FUNCTION_BLOCK "IMAC_MOTOR3"
TITLE = MOTOR 3
//--------------------------------------------------------------------------------
//SIEMENS AG     I&S IP PEP SN                        PSP-Element: D-09300081-E-E5
//--------------------------------------------------------------------------------
//History
//=======
//Date      Version  Description                        Author
//1997/06/09   0.6   Basic Edition                      Salge
//2004/11/05   1.0   Basic Edition converted to S7      Edelmann
//2004/12/07   1.1   Interface adapted                  Edelmann
//2004/12/07   1.1   Reset Outputs with feedbacks       Edelmann
//
//--------------------------------------------------------------------------------
//PLC:   >= S7-300
//--------------------------------------------------------------------------------
//Specification:   Refer "TECHFUNK.DOC"
//--------------------------------------------------------------------------------
//
//--------------------------------------------------------------------------------
//Called FC: FC90 "DELAYTIMER"
//           SFC20 "BLKMOV"
//--------------------------------------------------------------------------------
//
//--------------------------------------------------------------------------------
//Note:
//--------------------------------------------------------------------------------
// KNOW_HOW_PROTECT
AUTHOR : Sa_Edm
FAMILY : IMAC
NAME : Motor3
VERSION : 1.1


VAR_INPUT
  OBJ : INT ;
  RMOT : BOOL ;	//Local / Remote
  FWD : BOOL ;
  BACK : BOOL ;
  SLOW : BOOL ;
  FAST : BOOL ;
  FAUL : BOOL ;
  ACOM : WORD ;
  BLKO : BOOL ;
  PCONF : STRUCT
   LastRecord : INT  := 100;
   Pointer1stRecord : STRUCT
    S7ID : BYTE  := B#16#10;	//ANY pointer: ID S7
    RepeatFactor : INT  := 104;	//ANY pointer: repeat factor
    Typ : BYTE  := B#16#2;	//ANY pointer: data typ =02 BYTE =04 WORD =05 INT =06 DWORD =07 DINT =08 REAL
    DBNo : INT  := 82;	//ANY pointer: DB number, zero if no DB
    MemoryArea : BYTE  := B#16#84;	//ANY pointer: Memory area =81 IN =82 OUT =83 M =84 DB =85 DI =86 L
    DWHigh : BYTE ;	//ANY pointer: DW highest byte
    DWX : INT ;	//ANY pointer: DW low / bit (address = byte *8 + bit)
   END_STRUCT ;
  END_STRUCT ;
END_VAR
VAR_OUTPUT
  MFWD : BOOL ;
  MBAC : BOOL ;
  MSLO : BOOL ;
  MFAS : BOOL ;
  MSTO : BOOL ;
  STAT : WORD ;
  OSSTAT : WORD ;	//Status for OS
  OSALARM : WORD ;	//Alarms for OS
END_VAR
VAR_IN_OUT
  OSCOM : WORD ;
END_VAR
VAR
  Motor3 : STRUCT
   System : WORD ;
   CmdOS : WORD ;
   MirrorCmdOS : WORD ;
   Test : WORD ;
   AlarmOS : WORD ;
   StatusOS : WORD ;
   SysStatusOS : WORD ;
   Status1 : WORD ;
   Status2 : WORD ;
   Status3 : BYTE ;
   InputEdges : BYTE ;
   AutoEdges : WORD ;
   DataTimeExtFault : STRUCT
    StartTime : DINT ;
    StartEdge : BOOL ;
   END_STRUCT ;
   DataTimeFeedback : STRUCT
    StartTime : DINT ;
    StartEdge : BOOL ;
   END_STRUCT ;
   DataTimeActFault : STRUCT
    StartTime : DINT ;
    StartEdge : BOOL ;
   END_STRUCT ;
   DataTimeAutoAl : STRUCT
    StartTime : DINT ;
    StartEdge : BOOL ;
   END_STRUCT ;
   DataTimeRestart : STRUCT
    StartTime : DINT ;
    StartEdge : BOOL ;
   END_STRUCT ;
   DataTimeChgSF : STRUCT
    StartTime : DINT ;
    StartEdge : BOOL ;
   END_STRUCT ;
   DataTimeChgFS : STRUCT
    StartTime : DINT ;
    StartEdge : BOOL ;
   END_STRUCT ;
   DataTimeChgDirec : STRUCT
    StartTime : DINT ;
    StartEdge : BOOL ;
   END_STRUCT ;
   PCONF : STRUCT
    Modeswitches : STRUCT
     M0_ConstantOut : BOOL ;	// Constant Output MST1 MST2 MSTO (1); Feedback depended Output Anst. (0)
     M1_AutoManLoc : BOOL ;	// AUTO/ MANUAL/ LOCAL (1); MANUAL/ LOCAL (0)
     M2_NoActFeedFault : BOOL ;	// No Action- and Non-Feedback fault(1),
     M3_NoStopIfFault : BOOL ;	// No Stop-Signal if Failure occurs (1)
     M4_RestrtAftBlack : BOOL ;	// Restart after Blackout (1)
     M5_ResetOSonly : BOOL ;	// Reset Alarm only with RESET from OS (1); RESET and START/STOP-Command (0)
     sw06 : BOOL ;
     M7_ChgSFviaStop : BOOL ;	// Change from Slow->Fast via STOP(1)
     M8_ChgFSviaStop : BOOL ;	// Change from Fast->Slow via STOP(1)
     M9_StopIfAutoFail : BOOL ;	// Direct Stop if Auto Failure (1)
     M10_ExtFaultNC : BOOL ;
     sw11 : BOOL ;
     sw12 : BOOL ;
     sw13 : BOOL ;
     sw14 : BOOL ;
     sw15 : BOOL ;	//
    END_STRUCT ;
    DlyTExtFault : TIME ;	// Setpoint external fault delay
    DlyTFeedback : TIME ;	// Setpoint feedback fault delay
    DlyTActFault : TIME ;	// Setpoint Action Fault delay
    DlyTAutoAl : TIME ;	// Setpoint auto alarm delay
    DlyTRestart : TIME ;	// Setpoint restart after blackout delay
    DlyTChgSF : TIME ;	// Setpoint Waiting Delay Slow->Fast
    DlyTChgFS : TIME ;	// Setpoint Waiting Delay Fast->Slow
    DlyTChgDirec : TIME ;	// Setpoint change direction
   END_STRUCT ;
  END_STRUCT ;
  siFailRR : INT ;	//Failure blockmove read record
  siFailWR : INT ;	//Failure blockmove write record
END_VAR
VAR_TEMP
  M_200_0 : BOOL ;
  tbCmdManual : BOOL ;
  tbCmdAuto : BOOL ;
  M_200_3 : BOOL ;
  M_200_4 : BOOL ;
  M_200_5 : BOOL ;
  M_200_6 : BOOL ;
  M_200_7 : BOOL ;
  tbCmdStartR1 : BOOL ;
  tbCmdStartR2 : BOOL ;
  tbCmdStartL1 : BOOL ;
  tbCmdStartL2 : BOOL ;
  tbCmdStop : BOOL ;
  M_201_5 : BOOL ;
  M_201_6 : BOOL ;
  tbCmdReset : BOOL ;
  M_202_0 : BOOL ;
  M_202_1 : BOOL ;
  M_202_2 : BOOL ;
  M_202_3 : BOOL ;
  M_202_4 : BOOL ;
  M_202_5 : BOOL ;
  M_202_6 : BOOL ;
  M_202_7 : BOOL ;
  M_203_0 : BOOL ;
  M_203_1 : BOOL ;
  tbAutoFailInput : BOOL ;
  tbCmdLock : BOOL ;
  tbEmergencyOff : BOOL ;
  M_203_5 : BOOL ;
  M_203_6 : BOOL ;
  M_203_7 : BOOL ;
  M_204_0 : BOOL ;
  M_204_1 : BOOL ;
  M_204_2 : BOOL ;
  M_204_3 : BOOL ;
  M_204_4 : BOOL ;
  M_204_5 : BOOL ;
  M_204_6 : BOOL ;
  M_204_7 : BOOL ;
  tbCommandStartR1Auto : BOOL ;
  tbCommandStopAuto : BOOL ;
  tbAutoFailInputPulse : BOOL ;
  M_205_3 : BOOL ;
  M_205_4 : BOOL ;
  tbCommandStartR2Auto : BOOL ;
  tbCommandStartL1Auto : BOOL ;
  tbCommandStartL2Auto : BOOL ;
  tbRemoteLocal : BOOL ;
  tbRunningFWD : BOOL ;
  tbFault : BOOL ;
  tbBlackout : BOOL ;
  tbRunningBack : BOOL ;
  tbRunningSlow : BOOL ;
  tbRunningFast : BOOL ;
  M_206_7 : BOOL ;
  M_207_0 : BOOL ;
  M_207_1 : BOOL ;
  M_207_2 : BOOL ;
  M_207_3 : BOOL ;
  M_207_4 : BOOL ;
  M_207_5 : BOOL ;
  M_207_6 : BOOL ;
  M_207_7 : BOOL ;
  tbStateFWDFast : BOOL ;
  tbStateBackSlow : BOOL ;
  tbStateBackFast : BOOL ;
  M_208_3 : BOOL ;
  M_208_4 : BOOL ;
  M_208_5 : BOOL ;
  M_208_6 : BOOL ;
  M_208_7 : BOOL ;
  tbStateFWDSlow : BOOL ;
  tbStateLocal : BOOL ;
  tbStateManual : BOOL ;
  tbStateAuto : BOOL ;
  tbStateFault : BOOL ;
  tbStateBlackout : BOOL ;
  M_209_6 : BOOL ;
  M_209_7 : BOOL ;
  M_210_0 : BOOL ;
  M_210_1 : BOOL ;
  M_210_2 : BOOL ;
  M_210_3 : BOOL ;
  M_210_4 : BOOL ;
  M_210_5 : BOOL ;
  M_210_6 : BOOL ;
  M_210_7 : BOOL ;
  M_211_0 : BOOL ;
  M_211_1 : BOOL ;
  M_211_2 : BOOL ;
  M_211_3 : BOOL ;
  M_211_4 : BOOL ;
  M_211_5 : BOOL ;
  M_211_6 : BOOL ;
  M_211_7 : BOOL ;
  M_212_0 : BOOL ;
  M_212_1 : BOOL ;
  M_212_2 : BOOL ;
  M_212_3 : BOOL ;
  M_212_4 : BOOL ;
  M_212_5 : BOOL ;
  M_212_6 : BOOL ;
  M_212_7 : BOOL ;
  M_213_0 : BOOL ;
  M_213_1 : BOOL ;
  M_213_2 : BOOL ;
  M_213_3 : BOOL ;
  M_213_4 : BOOL ;
  M_213_5 : BOOL ;
  M_213_6 : BOOL ;
  M_213_7 : BOOL ;
  tbNonFeedbackTimer : BOOL ;
  tbNonFeedbackAlarm : BOOL ;
  tbActionTimer : BOOL ;
  tbActionAlarm : BOOL ;
  tbAutoTimer : BOOL ;
  tbAutoAlarm : BOOL ;
  tbBlackoutStartF1 : BOOL ;
  tbRestartAfterBlackout : BOOL ;
  tbOutStartF1 : BOOL ;
  tbOutStop : BOOL ;
  tbLocal : BOOL ;
  tbOutManual : BOOL ;
  tbOutAuto : BOOL ;
  M_215_5 : BOOL ;
  tbExternalFault : BOOL ;
  tbFaultInputAlarm : BOOL ;
  tbBlackoutStartB1 : BOOL ;
  tbOutStartB2 : BOOL ;
  tbBlackoutStartB2 : BOOL ;
  tbOutputMFWD : BOOL ;
  tbOutputMBAC : BOOL ;
  tbOutputMSLO : BOOL ;
  tbOutputMFAS : BOOL ;
  tbOutputMSTO : BOOL ;
  M_217_0 : BOOL ;
  tbOutChangeToStartF1 : BOOL ;
  tbOutChangeToStartF2 : BOOL ;
  tbOutChangeToStartB1 : BOOL ;
  tbOutChangeToStartB2 : BOOL ;
  tbOutStartF2 : BOOL ;
  tbBlackoutStartF2 : BOOL ;
  tbOutStartB1 : BOOL ;
  tbLocaltoRemote : BOOL ;
  M_218_1 : BOOL ;
  M_218_2 : BOOL ;
  M_218_3 : BOOL ;
  M_218_4 : BOOL ;
  M_218_5 : BOOL ;
  M_218_6 : BOOL ;
  M_218_7 : BOOL ;
  tbWaitingTime1_2 : BOOL ;
  tbWaitingTime2_1 : BOOL ;
  tbChangeDirecTimer2_1 : BOOL ;
  M_219_3 : BOOL ;
  tbResetStopping : BOOL ;
  M_219_5 : BOOL ;
  M_219_6 : BOOL ;
  M_219_7 : BOOL ;
  M_220_0 : BOOL ;
  M_220_1 : BOOL ;
  M_220_2 : BOOL ;
  M_220_3 : BOOL ;
  M_220_4 : BOOL ;
  M_220_5 : BOOL ;
  M_220_6 : BOOL ;
  M_220_7 : BOOL ;
  M_221_0 : BOOL ;
  M_221_1 : BOOL ;
  M_221_2 : BOOL ;
  M_221_3 : BOOL ;
  M_221_4 : BOOL ;
  M_221_5 : BOOL ;
  M_221_6 : BOOL ;
  M_221_7 : BOOL ;
  P_currentRecord : ANY ;	//ANY pointer of the current record
END_VAR
BEGIN
NETWORK
TITLE =Calculation of current ANY pointer for reading /writing record
// ANY-pointer of current record
      L     #PCONF.Pointer1stRecord.S7ID;
      T     LB    22;
      L     #PCONF.Pointer1stRecord.Typ;
      T     LB    23;
      L     #PCONF.Pointer1stRecord.RepeatFactor;
      T     LW    24;
      L     #PCONF.Pointer1stRecord.DBNo;
      T     LW    26;
      L     #PCONF.Pointer1stRecord.MemoryArea;
      T     LB    28;
      L     #PCONF.Pointer1stRecord.DWHigh;
      T     LB    29;
      L     #PCONF.Pointer1stRecord.DWX;
      T     LW    30;

      L     #OBJ; //Check whether Obj within the range
      L     #PCONF.LastRecord;
      >I    ;
      SPB   cRcd;
      L     #OBJ;
      L     1;
      <I    ;
      SPB   cRcd;
      L     #OBJ;
cRcd: +     -1;
      L     #PCONF.Pointer1stRecord.RepeatFactor;
      *I    ;
      SLD   3; //DBW + DBX address of the current record
      L     LD    28;
      OD    ;
      T     LD    28; //DBWX part of ANY pointer "P_currentRecord"
NETWORK
TITLE =Read record

      CALL "BLKMOV" (
           SRCBLK                   := #P_currentRecord,
           RET_VAL                  := #siFailRR,
           DSTBLK                   := #Motor3);

NETWORK
TITLE =Read OS command

      L     #OSCOM; // Commands from OS
      T     LW     0;
      L     #Motor3.Status1; // Status stored
      T     LW    14;
      L     #Motor3.Status2; // Status stored
      T     LW    16;
      L     #Motor3.Status3; // Status stored
      T     LB    19;

      L     0; //Reset scratch  flags
      T     LW     6;
      T     LW    50;
      T     LW    52;
      T     LW    54;
NETWORK
TITLE =Formaloperanden Inputs

      U     #RMOT;
      =     #tbRemoteLocal; //Remote/Local
      U     #FWD;
      =     #tbRunningFWD; //Running foreward
      U     #BACK;
      =     #tbRunningBack; //Running back
      U     #SLOW;
      =     #tbRunningSlow; //Running slow
      U     #FAST;
      =     #tbRunningFast; //Running fast

      U     #Motor3.PCONF.Modeswitches.M10_ExtFaultNC;
      SPB   NC;
      U     #FAUL;
      =     #tbFault; //Fault
      SPA   GO;
NC:   UN    #FAUL;
      =     #tbFault; //Fault

GO:   L     #ACOM;
      T     LW     2; // Command From Automatic

      U     #BLKO;
      =     #tbBlackout; //Blackout

// ----Evaluate Pulsflags from Auto Commands----
      L     #Motor3.AutoEdges; //Stored Auto Command last cycle
      INVI  ; //Singlecomplement
      L     LW     2; //Command From Automatic
      T     #Motor3.AutoEdges;
      UW    ;
      T     LW     4; // Command  Pulseflags

// ----Evaluate Pulsflags from Inputs----
      L     #Motor3.InputEdges; //Stored Auto Command last cycle
      INVI  ; //Singlecomplement
      L     LB     6; //Inputs
      T     #Motor3.InputEdges;
      UW    ;
      T     LB    18; // Inputs Pulseflags
NETWORK
TITLE =Local-Manual- Auto

      UN    #tbRemoteLocal; // Not Remote
      =     #tbLocal; // LOCAL
      R     #tbOutManual; // MANUAL!
      R     #tbOutAuto; // AUTO!
      R     #tbOutChangeToStartF1; // Change to STARTF1!
      R     #tbOutChangeToStartF2; // Change to STARTF2!
      R     #tbOutChangeToStartB1; // Change to STARTB1!
      R     #tbOutChangeToStartB2; // Change to STARTB2!
      R     #tbOutStartF1; // STARTF1!
      R     #tbOutStartF2; // STARTF2!
      R     #tbOutStartB1; // STARTB1!
      R     #tbOutStartB2; // STARTB2!
      R     #tbOutStop; // STOP!
      R     #tbBlackoutStartF1; // BLACKOUT START F1
      R     #tbBlackoutStartF2; // BLACKOUT START F2
      R     #tbBlackoutStartB1; // BLACKOUT START B1
      R     #tbBlackoutStartB2; // BLACKOUT START B2
      R     #tbNonFeedbackTimer; // reset Non Feedback Timer
      R     #tbActionTimer; // reset Action Timer
      R     #tbAutoTimer; // reset Auto Timer
      R     #tbWaitingTime1_2; // reset Wating timer1->2
      R     #tbChangeDirecTimer2_1; // Change direction timer2->1
      R     #tbResetStopping; // reset Stopping


      SPB   E05;
      U     #Motor3.PCONF.Modeswitches.M1_AutoManLoc; // extra Automode ?
      SPB   MODE;
      S     #tbOutManual; //MANUAL!
      S     #tbOutAuto; // AUTO!
      SPA   E05;
MODE: U     #tbCmdManual; //Command Manual
      S     #tbOutManual; //MANUAL!
      R     #tbOutAuto; // AUTO!
      U     #tbCmdAuto; //Command Auto
      S     #tbOutAuto; // AUTO!
      R     #tbOutManual; // MANUAL!
      UN    #tbOutAuto; // AUTO!
      UN    #tbOutManual; // MANUAL!
      S     #tbOutManual; // MANUAL!
E05:  NOP   0;


NETWORK
TITLE =Commands
// SET Start forward 1 Command
      L     LW     0;
      U     #M_200_7;
      U     #tbCmdReset;
      O(    ;
      U     #tbCmdStartR1; //Command Start R1  OS Pulse
      U     #tbOutManual; //MANUAL!
      )     ;
      O(    ;
      U     #tbCommandStartR1Auto; //Command Start R1 Auto Pulse
      U     #tbOutAuto; //AUTO!
      )     ;
      S     #tbOutStartF1; //STARTF1!
      S     L     51.0; //STARTF1 Pulse

//SET Start Forward 2 Command
      O(    ;
      U     #tbCmdStartR2; //Command Start R2 OS Pulse
      U     #tbOutManual; //MANUAL!
      )     ;
      O(    ;
      U     #tbCommandStartR2Auto; //Command Start R2 Auto Pulse
      U     #tbOutAuto; //AUTO!
      )     ;
      S     #tbOutStartF2; //STARTF2!
      S     L     51.2; //STARTF2 Pulse

//SET Start BACK1 Command
      O(    ;
      U     #tbCmdStartL1; //Command Start L1  OS Pulse
      U     #tbOutManual; //MANUAL!
      )     ;
      O(    ;
      U     #tbCommandStartL1Auto; //Command Start L1 Auto Pulse
      U     #tbOutAuto; //AUTO!
      )     ;
      S     #tbOutStartB1; //STARTB1!
      S     L     51.3; //STARTF1 Pulse

//SET Start Back2 Command
      O(    ;
      U     #tbCmdStartL2; //Command Start L2 OS Pulse
      U     #tbOutManual; //MANUAL!
      )     ;
      O(    ;
      U     #tbCommandStartL2Auto; //Command Start L2 Auto Pulse | Corr: Edm, 08.12.04
      U     #tbOutAuto; //AUTO!
      )     ;
      S     #tbOutStartB2; //STARTB2!
      S     L     51.4; //STARTB2 Pulse

//SET Stop Command
      O(    ;
      U     #tbCmdStop; //Command Stop OS Pulse
      U     #tbOutManual; //MANUAL!
      )     ;
      O(    ;
      U     #tbCommandStopAuto; //Command Stop Auto Pulse
      U     #tbOutAuto; //AUTO!
      )     ;
      S     #tbOutStop; //STOP!
      S     L     51.1; //STOP Pulse
      R     #tbOutChangeToStartF1; //Change to STARTF1!
      R     #tbOutChangeToStartF2; //Change to STARTF2!
      R     #tbOutChangeToStartB1; //Change to STARTB1!
      R     #tbOutChangeToStartB2; //Change to STARTB2!

//Reset Alarms
      O     L     51.0; //STARTF1! Pulse
      O     L     51.2; //STARTF2! Pulse
      O     L     51.3; //STARTB1! Pulse
      O     L     51.4; //STARTB2! Pulse
      O     L     51.1; //STOP! Pulse
      U     #Motor3.PCONF.Modeswitches.M5_ResetOSonly; //Modeswitch Reset Alarm with Start/Stop
      O     #tbCmdReset; //Command RESET OS Pulse
      R     #tbFaultInputAlarm; //Fault Input Alarm
      R     #tbNonFeedbackAlarm; //Non Feedback Alarm
      R     #tbActionAlarm; //Action Alarm
      R     #tbActionTimer; //Edm, 08.12.04
      R     #tbAutoAlarm; //Auto Alarm

//Reset START ! if Failure
      O     #tbFaultInputAlarm; //Fault Input Alarm
      O     #tbNonFeedbackAlarm; //Non Feedback Alarm
      O     #tbActionAlarm; //Action Alarm
      O     #tbAutoAlarm; //Auto Alarm
      U     #tbOutStartF1; //STARTF1!
      U     L     51.0; //STARTF1 Pulse
      R     #tbOutStartF1; //STARTF1!
      R     L     51.0; //STARTF1 Pulse
      S     #tbOutStop; //STOP!

      O     #tbFaultInputAlarm; //Fault Input Alarm
      O     #tbNonFeedbackAlarm; //Non Feedback Alarm
      O     #tbActionAlarm; //Action Alarm
      O     #tbAutoAlarm; //Auto Alarm
      U     #tbOutStartF2; //STARTF2
      U     L     51.2; //STARTF2 Pulse
      R     #tbOutStartF2; //STARTF2
      R     L     51.2; //STARTF2 Pulse
      S     #tbOutStop; //STOP!

      O     #tbFaultInputAlarm; //Fault Input Alarm
      O     #tbNonFeedbackAlarm; //Non Feedback Alarm
      O     #tbActionAlarm; //Action Alarm
      O     #tbAutoAlarm; //Auto Alarm
      U     #tbOutStartB1; //STARTB1!
      U     L     51.3; //STARTB1 Pulse
      R     #tbOutStartB1; //STARTB1!
      R     L     51.3; //STARTB1 Pulse
      S     #tbOutStop; //STOP!

      O     #tbFaultInputAlarm; //Fault Input Alarm
      O     #tbNonFeedbackAlarm; //Non Feedback Alarm
      O     #tbActionAlarm; //Action Alarm
      O     #tbAutoAlarm; //Auto Alarm
      U     #tbOutStartB2; //STARTB2!
      U     L     51.4; //STARTB2 Pulse
      R     #tbOutStartB2; //STARTB2!
      R     L     51.4; //STARTB2 Pulse
      S     #tbOutStop; //STOP!

      U     #tbLocaltoRemote; //Local to Remote Pulse
      U     #tbRunningFWD; //Running foreward
      U     #tbRunningSlow; //Running slow
      UN    #tbOutStartF1; //STARTF1!
      UN    #tbOutStartF2; //STARTF2!
      UN    #tbOutStartB1; //STARTB1!
      UN    #tbOutStartB2; //STARTB2!
      UN    #tbOutStop; //STOP!
      S     #tbOutStartF1; //STARTF1!

      U     #tbLocaltoRemote; //Local to Remote Pulse
      U     #tbRunningFWD; //Running foreward
      U     #tbRunningFast; //Running fast
      UN    #tbOutStartF1; //STARTF1!
      UN    #tbOutStartF2; //STARTF2!
      UN    #tbOutStartB1; //STARTB1!
      UN    #tbOutStartB2; //STARTB2!
      UN    #tbOutStop; //STOP!
      S     #tbOutStartF2; //STARTF2!

      U     #tbLocaltoRemote; //Local to Remote Pulse
      U     #tbRunningBack; //Running back
      U     #tbRunningSlow; //Running slow
      UN    #tbOutStartF1; //STARTF1!
      UN    #tbOutStartF2; //STARTF2!
      UN    #tbOutStartB1; //STARTB1!
      UN    #tbOutStartB2; //STARTB2!
      UN    #tbOutStop; //STOP!
      S     #tbOutStartB1; //STARTB1!

      U     #tbLocaltoRemote; //Local to Remote Pulse
      U     #tbRunningBack; //Running back
      U     #tbRunningFast; //Running fast
      UN    #tbOutStartF1; //STARTF1!
      UN    #tbOutStartF2; //STARTF2!
      UN    #tbOutStartB1; //STARTB1!
      UN    #tbOutStartB2; //STARTB2!
      UN    #tbOutStop; //STOP!
      S     #tbOutStartB2; //STARTB2!
NETWORK
TITLE =Change Mode 1
//STOP F1,F2,B1,B2 after 0
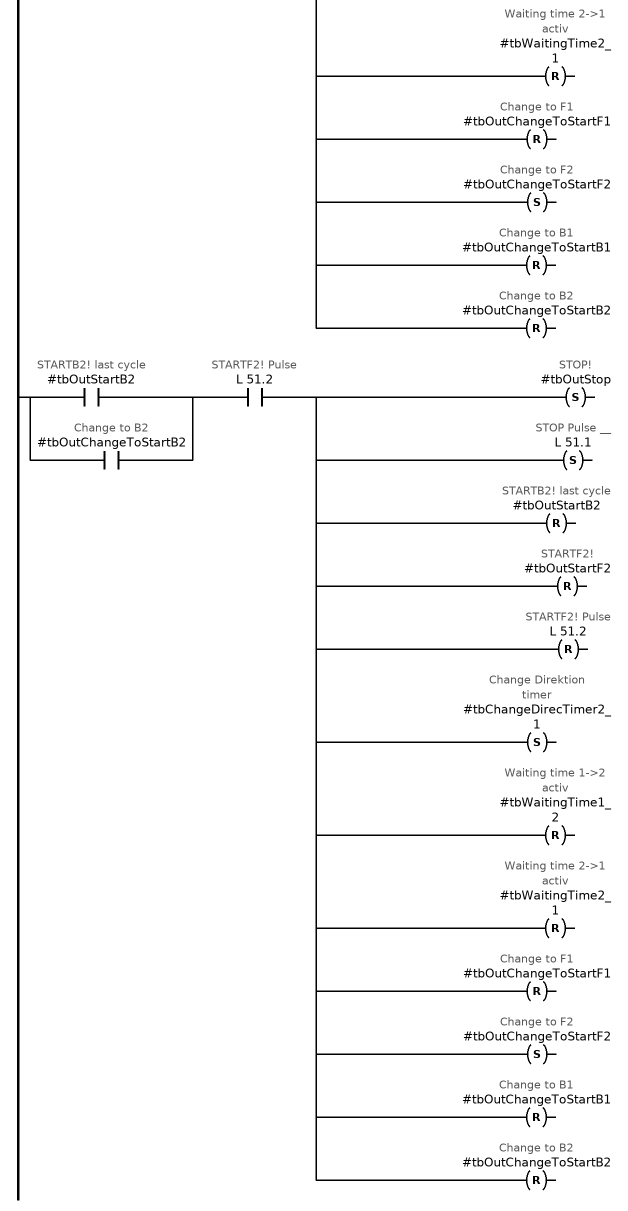
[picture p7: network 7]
      O     #tbOutStartF1; //STARTF1! Last cycle
      O     #tbOutStartF2; //STARTF2! Last cycle
      O     #tbOutStartB1; //STARTB1! Last cycle
      O     #tbOutStartB2; //STARTB2! Last cycle
      U     L     51.1; //STOP Pulse
      S     #tbChangeDirecTimer2_1; //Change Direktion timer
      R     #tbWaitingTime2_1; //Waiting time 2->1 activ
      R     #tbWaitingTime1_2; //Waiting time 1->2 activ

//Change from F1 to F2
      U     #tbOutStartF1; //STARTF1! last cycle
      U     L     51.2; //STARTF2! Pulse
      U     #Motor3.PCONF.Modeswitches.M7_ChgSFviaStop; //MOD Change from 1->2 via Stop
      S     #tbOutStop; //STOP!
      S     L     51.1; //STOP Pulse

      U     #tbOutStartF1; //STARTF1! last cycle
      U     L     51.2; //STARTF2! Pulse
      R     #tbOutStartF1; //STARTF1! last cycle
      R     #tbOutStartF2; //STARTF2!
      R     L     51.2; //STARTF2! Pulse
      S     #tbChangeDirecTimer2_1; //Change Direktion timer
      S     #tbWaitingTime1_2; //Waiting time 1->2 activ
      R     #tbWaitingTime2_1; //Waiting time 2->1 activ
      R     #tbOutChangeToStartF1; //Change to F1
      S     #tbOutChangeToStartF2; //Change to F2
      R     #tbOutChangeToStartB1; //Change to B1
      R     #tbOutChangeToStartB2; //Change to B2

//Change from F2 to F1
      U     #tbOutStartF2; //STARTF2! last cycle
      U     L     51.0; //STARTF1! Pulse
      U     #Motor3.PCONF.Modeswitches.M8_ChgFSviaStop; //MOD Change from 2->1 via Stop
      S     #tbOutStop; //STOP!
      S     L     51.1; //STOP Pulse

      U     #tbOutStartF2; //STARTF2! last cycle
      U     L     51.0; //STARTF1! Pulse
      R     #tbOutStartF2; //STARTF2! last cycle
      R     #tbOutStartF1; //STARTF1! _
      R     L     51.0; //STARTF1! Pulse
      S     #tbChangeDirecTimer2_1; //Change Direktion timer
      R     #tbWaitingTime1_2; //Waiting time 1->2 activ
      S     #tbWaitingTime2_1; //Waiting time 2->1 activ
      S     #tbOutChangeToStartF1; //Change to F1
      R     #tbOutChangeToStartF2; //Change to F2
      R     #tbOutChangeToStartB1; //Change to B1
      R     #tbOutChangeToStartB2; //Change to B2

//Change from B1 to B2
      U     #tbOutStartB1; //STARTB1! last cycle
      U     L     51.4; //STARTB2! Pulse
      U     #Motor3.PCONF.Modeswitches.M7_ChgSFviaStop; //MOD Change from 1->2 via Stop
      S     #tbOutStop; //STOP!
      S     L     51.1; //STOP Pulse

      U     #tbOutStartB1; //STARTB1! last cycle
      U     L     51.4; //STARTB2! Pulse
      R     #tbOutStartB1; //STARTB1! last cycle
      R     #tbOutStartB2; //STARTB2!
      R     L     51.4; //STARTB2! Pulse
      S     #tbChangeDirecTimer2_1; //Change Direktion timer
      S     #tbWaitingTime1_2; //Waiting time 1->2 activ
      R     #tbWaitingTime2_1; //Waiting time 2->1 activ
      R     #tbOutChangeToStartF1; //Change to F1
      R     #tbOutChangeToStartF2; //Change to F2
      R     #tbOutChangeToStartB1; //Change to B1
      S     #tbOutChangeToStartB2; //Change to B2

//Change from B2 to B1
      U     #tbOutStartB2; //STARTB2! last cycle
      U     L     51.3; //STARTB1! Pulse
      U     #Motor3.PCONF.Modeswitches.M8_ChgFSviaStop; //MOD Change from 2->1 via Stop
      S     #tbOutStop; //STOP!
      S     L     51.1; //STOP Pulse

      U     #tbOutStartB2; //STARTB2! last cycle
      U     L     51.3; //STARTB1! Pulse
      R     #tbOutStartB2; //STARTB2! last cycle
      R     #tbOutStartB1; //STARTB1! _
      R     L     51.3; //STARTB1! Pulse
      S     #tbChangeDirecTimer2_1; //Change Direktion timer
      R     #tbWaitingTime1_2; //Waiting time 1->2 activ
      S     #tbWaitingTime2_1; //Waiting time 2->1 activ
      R     #tbOutChangeToStartF1; //Change to F1
      R     #tbOutChangeToStartF2; //Change to F2
      S     #tbOutChangeToStartB1; //Change to B1
      R     #tbOutChangeToStartB2; //Change to B2

//=====================================================
//Change from F1 to B1
      U(    ;
      O     #tbOutStartF1; //STARTF1! last cycle
      O     #tbOutChangeToStartF1; //Change to F1
      )     ;
      U     L     51.3; //STARTB1! Pulse
      S     #tbOutStop; //STOP!
      S     L     51.1; //STOP Pulse
      R     #tbOutStartF1; //STARTF1! last cycle
      R     #tbOutStartB1; //STARTB1!
      R     L     51.3; //STARTB1! Pulse
      S     #tbChangeDirecTimer2_1; //Change Direktion timer
      R     #tbWaitingTime1_2; //Waiting time 1->2 activ
      R     #tbWaitingTime2_1; //Waiting time 2->1 activ
      R     #tbOutChangeToStartF1; //Change to F1
      R     #tbOutChangeToStartF2; //Change to F2
      S     #tbOutChangeToStartB1; //Change to B1
      R     #tbOutChangeToStartB2; //Change to B2

//Change from F2 to B1
      U(    ;
      O     #tbOutStartF2; //STARTF2! last cycle
      O     #tbOutChangeToStartF2; //Change to F2
      )     ;
      U     L     51.3; //STARTB1! Pulse
      S     #tbOutStop; //STOP!
      S     L     51.1; //STOP Pulse
      R     #tbOutStartF2; //STARTF2! last cycle
      R     #tbOutStartB1; //STARTB1!
      R     L     51.3; //STARTB1! Pulse
      S     #tbChangeDirecTimer2_1; //Change Direktion timer
      R     #tbWaitingTime1_2; //Waiting time 1->2 activ
      R     #tbWaitingTime2_1; //Waiting time 2->1 activ
      R     #tbOutChangeToStartF1; //Change to F1
      R     #tbOutChangeToStartF2; //Change to F2
      S     #tbOutChangeToStartB1; //Change to B1
      R     #tbOutChangeToStartB2; //Change to B2

//Change from F1 to B2
      U(    ;
      O     #tbOutStartF1; //STARTF1! last cycle
      O     #tbOutChangeToStartF1; //Change to F1
      )     ;
      U     L     51.4; //STARTB2! Pulse
      S     #tbOutStop; //STOP!
      S     L     51.1; //STOP Pulse
      R     #tbOutStartF1; //STARTF1! last cycle
      R     #tbOutStartB2; //STARTB2!
      R     L     51.4; //STARTB2! Pulse
      S     #tbChangeDirecTimer2_1; //Change Direktion timer
      R     #tbWaitingTime1_2; //Waiting time 1->2 activ
      R     #tbWaitingTime2_1; //Waiting time 2->1 activ
      R     #tbOutChangeToStartF1; //Change to F1
      R     #tbOutChangeToStartF2; //Change to F2
      R     #tbOutChangeToStartB1; //Change to B1
      S     #tbOutChangeToStartB2; //Change to B2

//Change from F2 to B2
      U(    ;
      O     #tbOutStartF2; //STARTF2! last cycle
      O     #tbOutChangeToStartF2; //Change to F2
      )     ;
      U     L     51.4; //STARTB2! Pulse
      S     #tbOutStop; //STOP!
      S     L     51.1; //STOP Pulse
      R     #tbOutStartF2; //STARTF2! last cycle
      R     #tbOutStartB2; //STARTB2!
      R     L     51.4; //STARTB2! Pulse
      S     #tbChangeDirecTimer2_1; //Change Direktion timer
      R     #tbWaitingTime1_2; //Waiting time 1->2 activ
      R     #tbWaitingTime2_1; //Waiting time 2->1 activ
      R     #tbOutChangeToStartF1; //Change to F1
      R     #tbOutChangeToStartF2; //Change to F2
      R     #tbOutChangeToStartB1; //Change to B1
      S     #tbOutChangeToStartB2; //Change to B2

//Change from B1 to F1
      U(    ;
      O     #tbOutStartB1; //STARTB1! last cycle
      O     #tbOutChangeToStartB1; //Change to B1
      )     ;
      U     L     51.0; //STARTF1! Pulse
      S     #tbOutStop; //STOP!
      S     L     51.1; //STOP Pulse
      R     #tbOutStartB1; //STARTB1! last cycle
      R     #tbOutStartF1; //STARTF1!
      R     L     51.0; //STARTF1! Pulse
      S     #tbChangeDirecTimer2_1; //Change Direktion timer
      R     #tbWaitingTime1_2; //Waiting time 1->2 activ
      R     #tbWaitingTime2_1; //Waiting time 2->1 activ
      S     #tbOutChangeToStartF1; //Change to F1
      R     #tbOutChangeToStartF2; //Change to F2
      R     #tbOutChangeToStartB1; //Change to B1
      R     #tbOutChangeToStartB2; //Change to B2

//Change from B2 to F1
      U(    ;
      O     #tbOutStartB2; //STARTB2! last cycle
      O     #tbOutChangeToStartB2; //Change to B2
      )     ;
      U     L     51.0; //STARTF1! Pulse
      S     #tbOutStop; //STOP!
      S     L     51.1; //STOP Pulse
      R     #tbOutStartB2; //STARTB2! last cycle
      R     #tbOutStartF1; //STARTF1!
      R     L     51.0; //STARTF1! Pulse
      S     #tbChangeDirecTimer2_1; //Change Direktion timer
      R     #tbWaitingTime1_2; //Waiting time 1->2 activ
      R     #tbWaitingTime2_1; //Waiting time 2->1 activ
      S     #tbOutChangeToStartF1; //Change to F1
      R     #tbOutChangeToStartF2; //Change to F2
      R     #tbOutChangeToStartB1; //Change to B1
      R     #tbOutChangeToStartB2; //Change to B2

//Change from B1 to F2
      U(    ;
      O     #tbOutStartB1; //STARTB1! last cycle
      O     #tbOutChangeToStartB1; //Change to B1
      )     ;
      U     L     51.2; //STARTF1! Pulse
      S     #tbOutStop; //STOP!
      S     L     51.1; //STOP Pulse
      R     #tbOutStartB1; //STARTB1! last cycle
      R     #tbOutStartF2; //STARTF2!
      R     L     51.2; //STARTF2! Pulse
      S     #tbChangeDirecTimer2_1; //Change Direktion timer
      R     #tbWaitingTime1_2; //Waiting time 1->2 activ
      R     #tbWaitingTime2_1; //Waiting time 2->1 activ
      R     #tbOutChangeToStartF1; //Change to F1
      S     #tbOutChangeToStartF2; //Change to F2
      R     #tbOutChangeToStartB1; //Change to B1
      R     #tbOutChangeToStartB2; //Change to B2

//Change from B2 to F2
      U(    ;
      O     #tbOutStartB2; //STARTB2! last cycle
      O     #tbOutChangeToStartB2; //Change to B2
      )     ;
      U     L     51.2; //STARTF2! Pulse
      S     #tbOutStop; //STOP!
      S     L     51.1; //STOP Pulse __
      R     #tbOutStartB2; //STARTB2! last cycle
      R     #tbOutStartF2; //STARTF2!
      R     L     51.2; //STARTF2! Pulse
      S     #tbChangeDirecTimer2_1; //Change Direktion timer
      R     #tbWaitingTime1_2; //Waiting time 1->2 activ
      R     #tbWaitingTime2_1; //Waiting time 2->1 activ
      R     #tbOutChangeToStartF1; //Change to F1
      S     #tbOutChangeToStartF2; //Change to F2
      R     #tbOutChangeToStartB1; //Change to B1
      R     #tbOutChangeToStartB2; //Change to B2
NETWORK
TITLE =Change Mode 2
//Change from STOP to 1
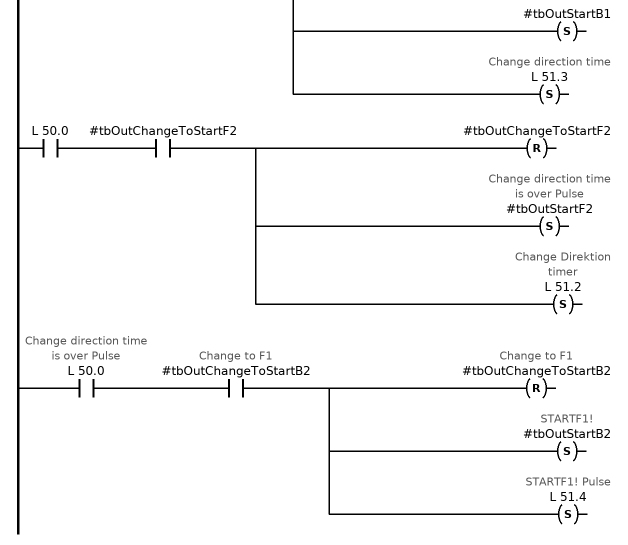
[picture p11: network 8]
      U     L     51.0; //STARTF1! Pulse
      U     #tbChangeDirecTimer2_1; //Change Direktion timer
      R     #tbOutStartF1; //STARTF1!
      R     L     51.0; //STARTF1! Pulse
      S     #tbOutChangeToStartF1; //Change to F1
      R     #tbOutChangeToStartF2; //Change to F2
      R     #tbOutChangeToStartB1; //Change to B1
      R     #tbOutChangeToStartB2; //Change to B2

      U     L     51.2; //STARTF2! Pulse
      U     #tbChangeDirecTimer2_1; //Change Direktion timer
      R     #tbOutStartF2; //STARTF2!
      R     L     51.2; //STARTF2! Pulse
      R     #tbOutChangeToStartF1; //Change to F1
      S     #tbOutChangeToStartF2; //Change to F2
      R     #tbOutChangeToStartB1; //Change to B1
      R     #tbOutChangeToStartB2; //Change to B2

      U     L     51.3; //STARTB1! Pulse
      U     #tbChangeDirecTimer2_1; //Change Direktion timer
      R     #tbOutStartB1; //STARTB1! _
      R     L     51.3; //STARTB1! Pulse
      R     #tbOutChangeToStartF1; //Change to F1
      R     #tbOutChangeToStartF2; //Change to F2
      S     #tbOutChangeToStartB1; //Change to B1
      R     #tbOutChangeToStartB2; //Change to B2

      U     L     51.4; //STARTB2! Pulse
      U     #tbChangeDirecTimer2_1; //Change Direktion timer
      R     #tbOutStartB2; //STARTB2!
      R     L     51.4; //STARTB2! Pulse
      R     #tbOutChangeToStartF1; //Change to F1
      R     #tbOutChangeToStartF2; //Change to F2
      R     #tbOutChangeToStartB1; //Change to B1
      S     #tbOutChangeToStartB2; //Change to B2

//Waiting Timer 1->2
      CALL "IMAC_DELAYTIMER" (
           XSTART                   := #tbWaitingTime1_2,//waiting time 1->2
           XTIME                    := #Motor3.PCONF.DlyTChgSF,
           YON                      := L     50.6,
           MEM                      := #Motor3.DataTimeChgSF);

      U     L     50.6; //waiting time 1->2 is over Pulse
      R     #tbWaitingTime1_2; //waiting time 1->2

      U     L     50.6;
      U     #tbOutChangeToStartF2;
      R     #tbOutChangeToStartF2;
      S     #tbOutStartF2; //waiting time 1->2 is over Pulse
      S     L     51.2; //Waiting time 1->2 activ
      R     #tbChangeDirecTimer2_1; //waiting time 1->2 is over Pulse

      U     L     50.6; //Change to F2
      U     #tbOutChangeToStartB2; //Change to F2
      R     #tbOutChangeToStartB2; //STARTF2!
      S     #tbOutStartB2; //STARTF2! Pulse
      S     L     51.4; //Change Direktion timer
      R     #tbChangeDirecTimer2_1; //waiting time 1->2 is over Pulse

//Waiting Timer 2->1
      CALL "IMAC_DELAYTIMER" (
           XSTART                   := #tbWaitingTime2_1,//waiting time 2->1
           XTIME                    := #Motor3.PCONF.DlyTChgFS,
           YON                      := L     50.7,
           MEM                      := #Motor3.DataTimeChgFS);

      U     L     50.7; //Change to B2
      R     #tbWaitingTime2_1; //STARTB2!

      U     L     50.7; //STARTB2! Pulse
      U     #tbOutChangeToStartF1; //Change Direktion timer
      R     #tbOutChangeToStartF1; //Timer
      S     #tbOutStartF1;
      S     L     51.0; //waiting time 2->1
      R     #tbChangeDirecTimer2_1;

      U     L     50.7;
      U     #tbOutChangeToStartB1;
      R     #tbOutChangeToStartB1; //waiting time 2->1 is over Pulse
      S     #tbOutStartB1; //Waiting time 2->1 activ
      S     L     51.3; //waiting time 2->1 is over Pulse
      R     #tbChangeDirecTimer2_1; //Change to F1

//Change direction timer
      CALL "IMAC_DELAYTIMER" (
           XSTART                   := #tbChangeDirecTimer2_1,//Change direction time
           XTIME                    := #Motor3.PCONF.DlyTChgDirec,
           YON                      := L     50.0,
           MEM                      := #Motor3.DataTimeChgDirec);

      U     L     50.0; //STARTF1!
      R     #tbChangeDirecTimer2_1; //STARTF1! Pulse

      U     L     50.0; //Change Direktion timer
      U     #tbOutChangeToStartF1; //waiting time 2->1 is over Pulse
      R     #tbOutChangeToStartF1; //Change to B1
      S     #tbOutStartF1; //Change to B1
      S     L     51.0; //STARTB1!

      U     L     50.0; //STARTB1! Pulse
      U     #tbOutChangeToStartB1; //Change Direktion timer
      R     #tbOutChangeToStartB1; //Timer
      S     #tbOutStartB1;
      S     L     51.3; //Change direction time

      U     L     50.0;
      U     #tbOutChangeToStartF2;
      R     #tbOutChangeToStartF2;
      S     #tbOutStartF2; //Change direction time is over Pulse
      S     L     51.2; //Change Direktion timer

      U     L     50.0; //Change direction time is over Pulse
      U     #tbOutChangeToStartB2; //Change to F1
      R     #tbOutChangeToStartB2; //Change to F1
      S     #tbOutStartB2; //STARTF1!
      S     L     51.4; //STARTF1! Pulse
NETWORK
TITLE =Restart after Blackout
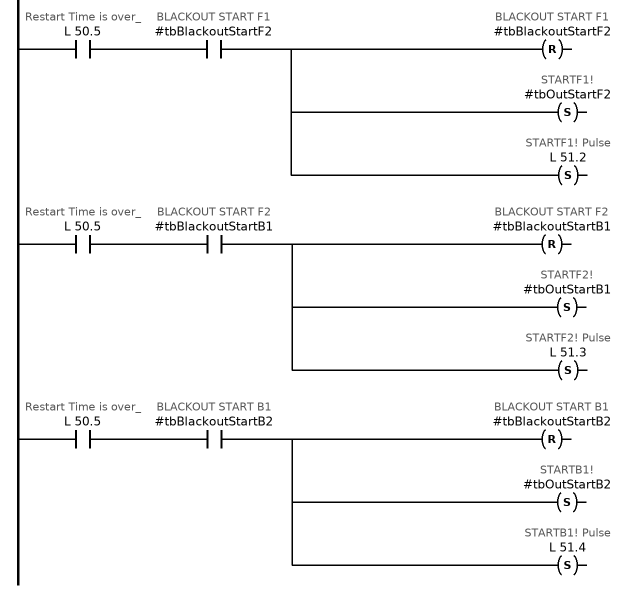
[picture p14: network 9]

      U     #tbBlackout; //Input Blackout
      U     #Motor3.PCONF.Modeswitches.M4_RestrtAftBlack; //Modeswitch Restart after Blackout
      U     #tbOutStartF1; //STARTF1!
      S     #tbBlackoutStartF1; //BLACKOUT START F1
      R     #tbBlackoutStartF2; //BLACKOUT START F2
      R     #tbBlackoutStartB1; //BLACKOUT START B1
      R     #tbBlackoutStartB2; //BLACKOUT START B2

      U     #tbBlackout; //Input Blackout
      U     #Motor3.PCONF.Modeswitches.M4_RestrtAftBlack; //Modeswitch Restart after Blackout
      U     #tbOutStartF2; //STARTF2!
      R     #tbBlackoutStartF1; //BLACKOUT START F1
      S     #tbBlackoutStartF2; //BLACKOUT START F2
      R     #tbBlackoutStartB1; //BLACKOUT START B1
      R     #tbBlackoutStartB2; //BLACKOUT START B2

      U     #tbBlackout; //Input Blackout
      U     #Motor3.PCONF.Modeswitches.M4_RestrtAftBlack; //Modeswitch Restart after Blackout
      U     #tbOutStartB1; //STARTB1!
      R     #tbBlackoutStartF1; //BLACKOUT START F1
      R     #tbBlackoutStartF2; //BLACKOUT START F2
      S     #tbBlackoutStartB1; //BLACKOUT START B1
      R     #tbBlackoutStartB2; //BLACKOUT START B2

      U     #tbBlackout; //Input Blackout
      U     #Motor3.PCONF.Modeswitches.M4_RestrtAftBlack; //Modeswitch Restart after Blackout
      U     #tbOutStartB2; //STARTB2!
      R     #tbBlackoutStartF1; //BLACKOUT START F1
      R     #tbBlackoutStartF2; //BLACKOUT START F2
      R     #tbBlackoutStartB1; //BLACKOUT START B1
      S     #tbBlackoutStartB2; //BLACKOUT START B2

      U     #tbBlackout; //Blackout
      R     #tbOutStartF1; //STARTF1!
      R     L     51.0; //STARTF1! Pulse
      R     #tbOutStartF2; //STARTF2!
      R     L     51.2; //STARTF2! Pulse
      R     #tbOutStartB1; //STARTB1!
      R     L     51.3; //STARTB1! Pulse
      R     #tbOutStartB2; //STARTB2!
      R     L     51.4; //STARTB2! Pulse
      R     #tbOutStop; //STOP!
      R     L     51.1; //STOP! Pulse

      U     L     51.1; //STOP!Pulse
      R     #tbBlackoutStartF1; //BLACKOUT START F1
      R     #tbBlackoutStartF2; //BLACKOUT START F2
      R     #tbBlackoutStartB1; //BLACKOUT START B1
      R     #tbBlackoutStartB2; //BLACKOUT START B2

      O     #tbBlackoutStartF1; //BLACKOUT START F1
      O     #tbBlackoutStartF2; //BLACKOUT START F2
      O     #tbBlackoutStartB1; //BLACKOUT START B1
      O     #tbBlackoutStartB2; //BLACKOUT START B2
      UN    #tbBlackout; //no Blackout
      =     #tbRestartAfterBlackout; //BLACKOUT START timer activ

//Restart timer
      CALL "IMAC_DELAYTIMER" (
           XSTART                   := #tbRestartAfterBlackout,//Restart time
           XTIME                    := #Motor3.PCONF.DlyTRestart,
           YON                      := L     50.5,
           MEM                      := #Motor3.DataTimeRestart);

      U     L     50.5;
      U     #tbBlackoutStartF1;
      R     #tbBlackoutStartF1;
      S     #tbOutStartF1;
      S     L     51.0;

      U     L     50.5; //Restart Time is over_
      U     #tbBlackoutStartF2; //BLACKOUT START F1
      R     #tbBlackoutStartF2; //BLACKOUT START F1
      S     #tbOutStartF2; //STARTF1!
      S     L     51.2; //STARTF1! Pulse

      U     L     50.5; //Restart Time is over_
      U     #tbBlackoutStartB1; //BLACKOUT START F2
      R     #tbBlackoutStartB1; //BLACKOUT START F2
      S     #tbOutStartB1; //STARTF2!
      S     L     51.3; //STARTF2! Pulse

      U     L     50.5; //Restart Time is over_
      U     #tbBlackoutStartB2; //BLACKOUT START B1
      R     #tbBlackoutStartB2; //BLACKOUT START B1
      S     #tbOutStartB2; //STARTB1!
      S     L     51.4; //STARTB1! Pulse
NETWORK
TITLE =Reset old states
//Reset old state (others in network "Commands")
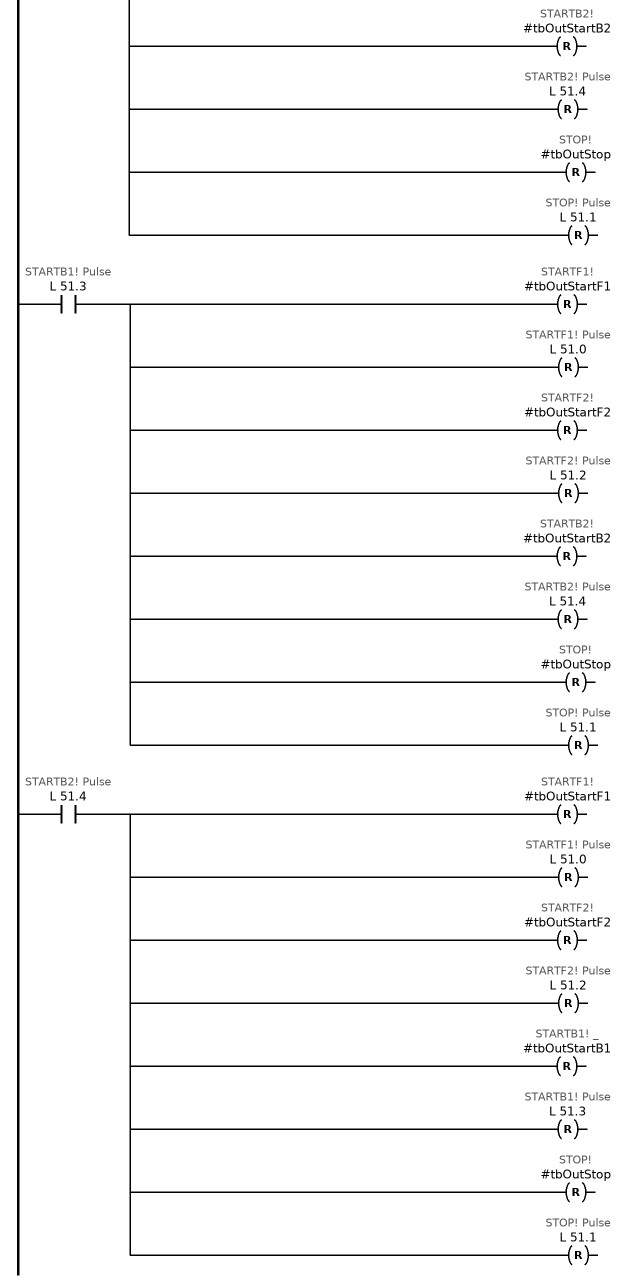
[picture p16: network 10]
      U     L     51.0; //STARTF1! Pulse
      R     #tbOutStartF2; //STARTF2!
      R     L     51.2; //STARTF2! Pulse
      R     #tbOutStartB1; //STARTB1! _
      R     L     51.3; //STARTB1! Pulse
      R     #tbOutStartB2; //STARTB2!
      R     L     51.4; //STARTB2! Pulse
      R     #tbOutStop; //STOP!
      R     L     51.1; //STOP! Pulse
      U     L     51.1; //STOP! Pulse
      R     #tbOutStartF1; //STARTF1!
      R     L     51.0; //STARTF1! Pulse
      R     #tbOutStartF2; //STARTF2!
      R     L     51.2; //STARTF2! Pulse
      R     #tbOutStartB1; //STARTB1! _
      R     L     51.3; //STARTB1! Pulse
      R     #tbOutStartB2; //STARTB2!
      R     L     51.4; //STARTB2! Pulse
      U     L     51.2; //STARTF2! Pulse
      R     #tbOutStartF1; //STARTF1!
      R     L     51.0; //STARTF1! Pulse
      R     #tbOutStartB1; //STARTB1! _
      R     L     51.3; //STARTB1! Pulse
      R     #tbOutStartB2; //STARTB2!
      R     L     51.4; //STARTB2! Pulse
      R     #tbOutStop; //STOP!
      R     L     51.1; //STOP! Pulse
      U     L     51.3; //STARTB1! Pulse
      R     #tbOutStartF1; //STARTF1!
      R     L     51.0; //STARTF1! Pulse
      R     #tbOutStartF2; //STARTF2!
      R     L     51.2; //STARTF2! Pulse
      R     #tbOutStartB2; //STARTB2!
      R     L     51.4; //STARTB2! Pulse
      R     #tbOutStop; //STOP!
      R     L     51.1; //STOP! Pulse
      U     L     51.4; //STARTB2! Pulse
      R     #tbOutStartF1; //STARTF1!
      R     L     51.0; //STARTF1! Pulse
      R     #tbOutStartF2; //STARTF2!
      R     L     51.2; //STARTF2! Pulse
      R     #tbOutStartB1; //STARTB1! _
      R     L     51.3; //STARTB1! Pulse
      R     #tbOutStop; //STOP!
      R     L     51.1; //STOP! Pulse
NETWORK
TITLE =Action Alarm

      U     #Motor3.PCONF.Modeswitches.M2_NoActFeedFault; //No Action and Feedback alarm
      SPB   E11;
      O     L     51.0; //STARTF1! Pulse
      O     L     51.2; //STARTF2! Pulse
      O     L     51.3; //STARTB1! Pulse
      O     L     51.4; //STARTB2! Pulse
      O     L     51.1; //STOP! Pulse
      S     #tbActionTimer; //Action Timer activ

//Action fault timer
      CALL "IMAC_DELAYTIMER" (
           XSTART                   := #tbActionTimer,//Action fault time activ
           XTIME                    := #Motor3.PCONF.DlyTActFault,
           YON                      := L     50.1,
           MEM                      := #Motor3.DataTimeActFault);

      U     L     50.1; //Action time is over
      S     #tbActionAlarm; //Action alarm
      U     L     50.1; //Action time is over
      UN    #Motor3.PCONF.Modeswitches.M3_NoStopIfFault; //Modeswitch Stop if alarm
      R     #tbOutStartF1; //StartF1!
      R     L     51.0; //Action time is over
      R     #tbOutStartF2; //Action alarm
      R     L     51.2; //Action time is over
      R     #tbOutStartB1; //Modswitch  Stop if alarm
      R     L     51.3; //STARTF1!
      R     #tbOutStartB2; //STARTF1! Pulse
      R     L     51.4; //STARTF2!

      O(    ; //STARTF2! Pulse
      U     #tbOutStartF1; //STARTB1!
      U     #tbRunningFWD; //STARTB1! Pulse
      U     #tbRunningSlow; //STARTB2!
      )     ; //STARTB2! Pulse
      O(    ;
      U     #tbOutStartF2; //STARTF1!
      U     #tbRunningFWD; //Running foreward
      U     #tbRunningFast; //Running slow
      )     ;
      O(    ;
      U     #tbOutStartB1; //STARTF2!
      U     #tbRunningBack; //Running foreward_
      U     #tbRunningSlow; //Running fast
      )     ;
      O(    ;
      U     #tbOutStartB2; //STARTB1! _
      U     #tbRunningBack; //Running back
      U     #tbRunningFast; //Running slow
      )     ;
      O(    ;
      U     #tbOutStop; //STARTB2!
      UN    #tbRunningFWD; //Running back
      UN    #tbRunningBack; //Running fast
      UN    #tbRunningSlow;
      UN    #tbRunningFast;
      )     ; //STOP!
      O     #tbBlackout; //Running foreward
      R     #tbActionTimer; //Running back
E11:  NOP   0;
NETWORK
TITLE =External Fault Alarm

      O     #tbOutAuto; //AUTO!
      O     #tbOutManual; //MANUAL!
      SPB   RMOT;
      U     #tbFault; //External Fault
      =     #tbFaultInputAlarm; //External Fault Alarm
      SPA   E12;
RMOT: U     #tbFault; //External Fault
      UN    #tbFaultInputAlarm; //External Fault Alarm
      UN    #tbBlackout; //Blackout
      =     #tbExternalFault; //Fault timer activ

//External fault timer
      CALL "IMAC_DELAYTIMER" (
           XSTART                   := #tbExternalFault,//External fault time activ
           XTIME                    := #Motor3.PCONF.DlyTExtFault,
           YON                      := L     50.2,
           MEM                      := #Motor3.DataTimeExtFault);

      U     L     50.2;
      S     #tbFaultInputAlarm;
      R     #tbOutStartF1; //Setpoint External Fault alarm d
      R     L     51.0; //Actual External Fault alarm del
      R     #tbOutStartF2;
      R     L     51.2; //Fault time over_
      R     #tbOutStartB1; //External Fault Alarm
      R     L     51.3; //STARTF1!
      R     #tbOutStartB2; //STARTF1! Pulse
      R     L     51.4; //STARTF2!
      S     #tbOutStop; //STARTF2! Pulse
      S     L     51.1; //STARTB1!
E12:  NOP   0;
NETWORK
TITLE =Non-Feedback alarm

      U     #Motor3.PCONF.Modeswitches.M2_NoActFeedFault; //Modeswitch No Action and Feedba
      SPB   E13;
      O(    ;
      ON    #tbRunningFWD; //Running foreward
      ON    #tbRunningSlow; //Running slow
      U     #tbOutStartF1; //STARTF1!
      )     ;
      O(    ;
      ON    #tbRunningFWD; //Running foreward_
      ON    #tbRunningFast; //Running fast
      U     #tbOutStartF2; //STARTF2!
      )     ;
      O(    ;
      ON    #tbRunningBack; //Running back
      ON    #tbRunningSlow; //Running slow
      U     #tbOutStartB1; //STARTB1! _
      )     ;
      O(    ;
      ON    #tbRunningBack; //Running back
      ON    #tbRunningFast; //Running fast
      U     #tbOutStartB2; //STARTB2!
      )     ;
      O(    ;
      O     #tbRunningFWD; //Running foreward
      O     #tbRunningBack; //Running back
      O     #tbRunningSlow; //Running slow
      O     #tbRunningFast; //Running fast
      U     #tbOutStop; //STOP!
      )     ;
      UN    #tbActionTimer; //no Action Timer activ
      UN    #tbActionAlarm; //no Action alarm
      UN    #tbExternalFault; //no Fault timer activ
      UN    #tbFaultInputAlarm; //no External Fault Alarm
      UN    #tbBlackout; //no Blackout
      =     #tbNonFeedbackTimer; //Non -Feedback Timer activ

//Non -Feedback timer
      CALL "IMAC_DELAYTIMER" (
           XSTART                   := #tbNonFeedbackTimer,//Non -Feedback Timer activ
           XTIME                    := #Motor3.PCONF.DlyTFeedback,
           YON                      := L     50.3,
           MEM                      := #Motor3.DataTimeFeedback);

      U     L     50.3;
      S     #tbNonFeedbackAlarm;
      U     L     50.3; //Setpoint Non Feedback alarm dela
      UN    #Motor3.PCONF.Modeswitches.M3_NoStopIfFault;
      R     #tbOutStartF1;
      R     L     51.0; //Non -Feedback time is over
      R     #tbOutStartF2; //Non -Feedback alarm
      R     L     51.2; //Non -Feedback time is over
      R     #tbOutStartB1; //Modswitch  Stop iif alarm
      R     L     51.3; //STARTF1!
      R     #tbOutStartB2; //STARTF1! Pulse
      R     L     51.4; //STARTF2!
      S     #tbOutStop; //STARTF2! Pulse
      S     L     51.1; //STARTB1!
E13:  NOP   0;


NETWORK
TITLE =Auto Failure

      UN    #tbOutAuto; //not in AUTO! Mode
      SPB   E14;
      U     #tbAutoFailInputPulse; //Auto failure Input pulse
      S     #tbAutoTimer; //Auto failure Timer activ
      UN    #tbAutoFailInput; //Auto failure Input
      R     #tbAutoTimer; //Auto failure Timer activ

//Auto Timer
      CALL "IMAC_DELAYTIMER" (
           XSTART                   := #tbAutoTimer,//Auto timer Timer activ
           XTIME                    := #Motor3.PCONF.DlyTAutoAl,
           YON                      := L     50.4,
           MEM                      := #Motor3.DataTimeAutoAl);

      U     L     50.4;
      S     #tbAutoAlarm;
      R     #tbOutStartF1;
      R     L     51.0;
      R     #tbOutStartF2;
      R     L     51.2; //Auto failure time is over
      R     #tbOutStartB1; //Auto failure alarm
      R     L     51.3; //STARTF1!
      R     #tbOutStartB2; //STARTF1! Pulse
      R     L     51.4; //STARTF2!
      S     #tbOutStop; //STARTF2! Pulse
      S     L     51.1; //STARTB1!
E14:  NOP   0;
NETWORK
TITLE =Automatic States
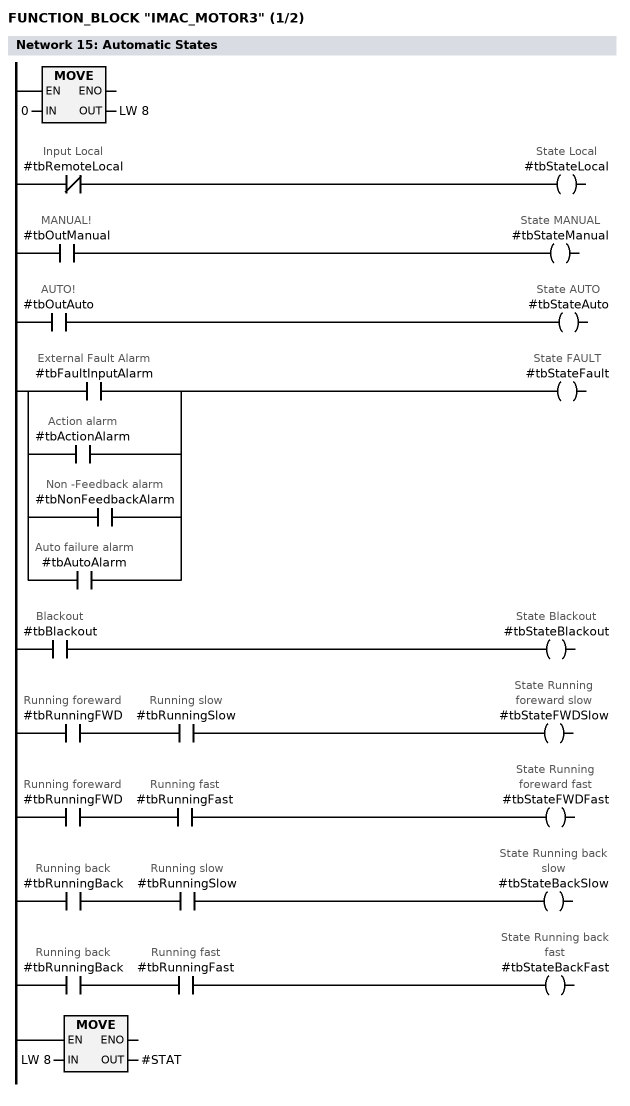
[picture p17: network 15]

      L     0;
      T     LW     8;

      UN    #tbRemoteLocal; //Input Local
      =     #tbStateLocal; //State Local
      U     #tbOutManual; //MANUAL!
      =     #tbStateManual; //State MANUAL
      U     #tbOutAuto; //AUTO!
      =     #tbStateAuto; //State AUTO
      O     #tbFaultInputAlarm; //External Fault Alarm
      O     #tbActionAlarm; //Action alarm
      O     #tbNonFeedbackAlarm; //Non -Feedback alarm
      O     #tbAutoAlarm; //Auto failure alarm
      =     #tbStateFault; //State FAULT
      U     #tbBlackout; //Blackout
      =     #tbStateBlackout; //State Blackout
      U     #tbRunningFWD; //Running foreward
      U     #tbRunningSlow; //Running slow
      =     #tbStateFWDSlow; //State Running foreward slow
      U     #tbRunningFWD; //Running foreward
      U     #tbRunningFast; //Running fast
      =     #tbStateFWDFast; //State Running foreward fast
      U     #tbRunningBack; //Running back
      U     #tbRunningSlow; //Running slow
      =     #tbStateBackSlow; //State Running back slow
      U     #tbRunningBack; //Running back
      U     #tbRunningFast; //Running fast
      =     #tbStateBackFast; //State Running back fast

      L     LW     8; // State To Automatic
      T     #STAT;
NETWORK
TITLE =Lock/ Emergency Off
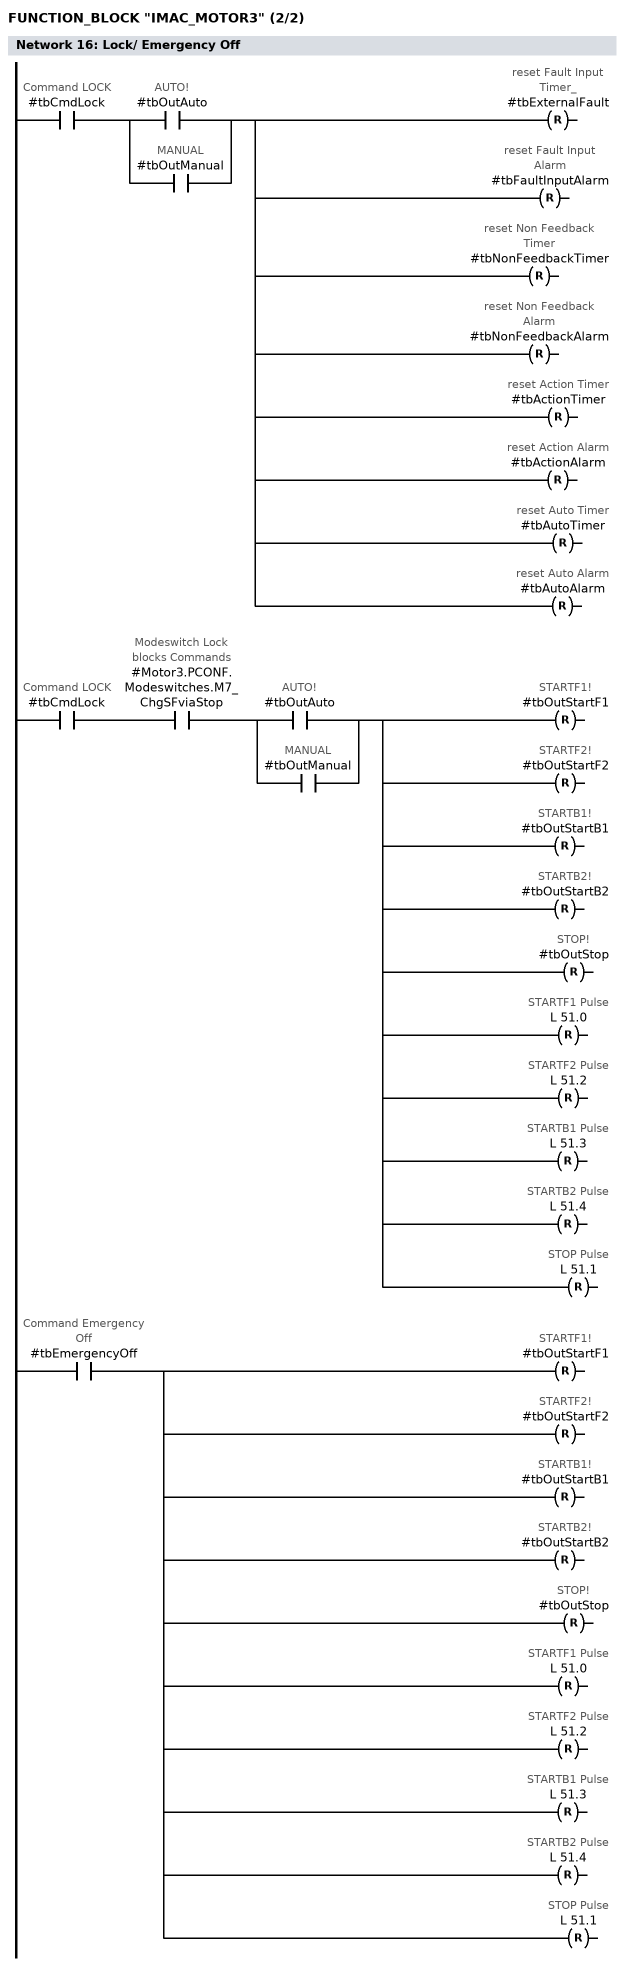
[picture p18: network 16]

      U     #tbCmdLock; //Command LOCK
      U(    ;
      O     #tbOutAuto; //AUTO!
      O     #tbOutManual; //MANUAL
      )     ;
      R     #tbExternalFault; //reset Fault Input Timer_
      R     #tbFaultInputAlarm; //reset Fault Input Alarm
      R     #tbNonFeedbackTimer; //reset Non Feedback Timer
      R     #tbNonFeedbackAlarm; //reset Non Feedback Alarm
      R     #tbActionTimer; //reset Action Timer
      R     #tbActionAlarm; //reset Action Alarm
      R     #tbAutoTimer; //reset Auto Timer
      R     #tbAutoAlarm; //reset Auto Alarm

      U     #tbCmdLock; //Command LOCK
      U     #Motor3.PCONF.Modeswitches.M7_ChgSFviaStop; //Modeswitch Lock blocks Commands
      U(    ;
      O     #tbOutAuto; //AUTO!
      O     #tbOutManual; //MANUAL
      )     ;
      R     #tbOutStartF1; //STARTF1!
      R     #tbOutStartF2; //STARTF2!
      R     #tbOutStartB1; //STARTB1!
      R     #tbOutStartB2; //STARTB2!
      R     #tbOutStop; //STOP!
      R     L     51.0; //STARTF1 Pulse
      R     L     51.2; //STARTF2 Pulse
      R     L     51.3; //STARTB1 Pulse
      R     L     51.4; //STARTB2 Pulse
      R     L     51.1; //STOP Pulse

//Emergency Off
      U     #tbEmergencyOff; //Command Emergency Off
      R     #tbOutStartF1; //STARTF1!
      R     #tbOutStartF2; //STARTF2!
      R     #tbOutStartB1; //STARTB1!
      R     #tbOutStartB2; //STARTB2!
      R     #tbOutStop; //STOP!
      R     L     51.0; //STARTF1 Pulse
      R     L     51.2; //STARTF2 Pulse
      R     L     51.3; //STARTB1 Pulse
      R     L     51.4; //STARTB2 Pulse
      R     L     51.1; //STOP Pulse
NETWORK
TITLE =Output

      U     #tbOutStop; //STOP!
      U     L     51.1; //STOP! Pulse
      R     #tbOutputMFWD; //Output MFWD foreward
      R     #tbOutputMBAC; //Output MBAC back
      R     #tbOutputMSLO; //Output MSLO slow
      R     #tbOutputMFAS; //Output MFAS fast
      S     #tbOutputMSTO; //Output MSTO stop

      U     #tbOutStartF1; //STARTF1!
      U     L     51.0; //STARTF1! Pulse
      S     #tbOutputMFWD; //Output MFWD foreward
      R     #tbOutputMBAC; //Output MBAC back
      S     #tbOutputMSLO; //Output MSLO slow
      R     #tbOutputMFAS; //Output MFAS fast
      R     #tbOutputMSTO; //Output MSTO stop

      U     #tbOutStartF2; //STARTF2!
      U     L     51.2; //STARTF2! Pulse
      S     #tbOutputMFWD; //Output MFWD foreward
      R     #tbOutputMBAC; //Output MBAC back
      R     #tbOutputMSLO; //Output MSLO slow
      S     #tbOutputMFAS; //Output MFAS fast
      R     #tbOutputMSTO; //Output MSTO stop

      U     #tbOutStartB1; //STARTB1!
      U     L     51.3; //STARTB1! Pulse
      R     #tbOutputMFWD; //Output MFWD foreward
      S     #tbOutputMBAC; //Output MBAC back
      S     #tbOutputMSLO; //Output MSLO slow
      R     #tbOutputMFAS; //Output MFAS fast
      R     #tbOutputMSTO; //Output MSTO stop

      U     #tbOutStartB2; //STARTB2!
      U     L     51.4; //STARTB2! Pulse
      R     #tbOutputMFWD; //Output MFWD foreward
      S     #tbOutputMBAC; //Output MBAC back
      R     #tbOutputMSLO; //Output MSLO slow
      S     #tbOutputMFAS; //Output MFAS fast
      R     #tbOutputMSTO; //Output MSTO stop

      UN    #tbOutStartF1; //STARTF1!
      UN    #tbOutStartF2; //STARTF2!
      R     #tbOutputMFWD; //Output MFWD foreward

      UN    #tbOutStartB1; //STARTB1! _
      UN    #tbOutStartB2; //STARTB2!
      R     #tbOutputMBAC; //Output MBAC back

      UN    #tbOutStartF1; //STARTF1!
      UN    #tbOutStartB1; //STARTB1! _
      R     #tbOutputMSLO; //Output MSLO slow

      UN    #tbOutStartF2; //STARTF2!
      UN    #tbOutStartB2; //STARTB2!
      R     #tbOutputMFAS; //Output MFAS fast

      UN    #tbRunningFWD; //Running foreward
      UN    #tbRunningBack; //Running back
      UN    #tbRunningSlow; //Running slow
      UN    #tbRunningFast; //Running fast
      UN    L     51.1; //STOP! Pulse
      ON    #tbOutStop; //STOP1!
      R     #tbOutputMSTO; //Output MSTO

      U     #Motor3.PCONF.Modeswitches.M0_ConstantOut;
      SPB   Out;
      U     #tbRunningFWD; //Running foreward
      R     #tbOutputMFWD;
      U     #tbRunningBack; //Running back
      R     #tbOutputMBAC; //Output back
      U     #tbRunningSlow; //Running slow
      R     #tbOutputMSLO; //Output slow
      U     #tbRunningFast; //Running fast
      R     #tbOutputMFAS; //Output fast

Out:  U     #tbOutputMFWD; //Output foreward
      =     #MFWD;
      U     #tbOutputMBAC; //Output back
      =     #MBAC;
      U     #tbOutputMSLO; //Output slow
      =     #MSLO;
      U     #tbOutputMFAS; //Output fast
      =     #MFAS;
      U     #tbOutputMSTO; //Output stop
      =     #MSTO;
NETWORK
TITLE =Combinate States
//----Alarms----
      U     #tbCmdLock; //Command LOCK
      U(    ;
      O     #tbOutAuto; //AUTO!
      O     #tbOutManual; //MANUAL
      )     ;
      L     6; //Lock
      SPB   COD1;
      U     #tbEmergencyOff; //Emergency Off
      L     7;
      SPB   COD1;
      UN    #tbFaultInputAlarm; //External Fault Alarm
      UN    #tbActionAlarm; //Action alarm
      UN    #tbNonFeedbackAlarm; //Non -Feedback alarm
      UN    #tbAutoAlarm; //Auto failure alarm
      UN    #tbBlackout; //Input Blackout
      L     1; //Normal
      SPB   COD1;
      U     #tbFaultInputAlarm; //External Fault Alarm
      L     2;
      SPB   COD1;
      U     #tbAutoAlarm; //Auto failure alarm
      L     3;
      SPB   COD1;
      U     #tbActionAlarm; //Action alarm
      L     4;
      SPB   COD1;
      U     #tbNonFeedbackAlarm; //Non -Feedback alarm
      L     5;
      SPB   COD1;
      U     #tbBlackout; //Input Blackout
      L     8;
      SPB   COD1;

      L     0; //Undefined
COD1: T     LW    10; //States to OS


//Status to OS

      O     #BLKO; //Backout
      O     #tbRestartAfterBlackout; // BLACKOUT START timer active
      L     11; //Blackout
      SPB   COD2;
      U     #tbRunningFWD; //Running foreward
      U     #tbRunningSlow; //Running slow
      L     1; //Running1
      SPB   COD2;
      U     #tbRunningFWD; //Running foreward
      U     #tbRunningFast; //Running fast
      L     2; //Running2
      SPB   COD2;
      U     #tbRunningBack; //Running back
      U     #tbRunningSlow; //Running slow
      L     3; //Running back slow in Local
      SPB   COD2;
      U     #tbRunningBack; //Running back
      U     #tbRunningFast; //Running fast
      L     4; //Running back fast in Local
      SPB   COD2;
//     U     #tbAuto; // AUTO!
//     UN    #tbStartTact; // START Timer activ
//     UN    #tbExtFaultA; // External Fault Alarm
//     UN    #tbActionA; // Action alarm
//     UN    #tbNonFeedbackA; // Non -Feedback alarm
//     UN    #tbAutoA; // Auto failure alarm
//     UN    #tbBlackout; // Input Blackout
//     U     #tbAutoStbyCtrl; //Standbycontrol active
//     L     5; //Standby
//     SPB   COD2;
      U     #tbOutputMFWD; //Output MFWD foreward
      U     #tbOutputMSLO; //Output MSLO slow
      UN    #tbRunningFWD; //Running foreward
      UN    #tbRunningSlow; //Running slow
      L     6; //Starting1
      SPB   COD2;
      U     #tbOutputMFWD; //Output MFWD foreward
      U     #tbOutputMFAS; //Output MFAS fast
      UN    #tbRunningFWD; //Running foreward
      UN    #tbRunningFast; //Running fast
      L     7; //Starting2
      SPB   COD2;
      U     #tbOutputMBAC; //Output MBAC back
      U     #tbOutputMSLO; //Output MSLO slow
      UN    #tbRunningBack; //Running back
      UN    #tbRunningSlow; //Running slow
      L     8; //Starting3
      SPB   COD2;
      U     #tbOutputMBAC; //Output MBAC back
      U     #tbOutputMFAS; //Output MFAS fast
      UN    #tbRunningBack; //Running back
      UN    #tbRunningFast; //Running fast
      L     9; //Starting3
      SPB   COD2;
      UN    #tbRunningFWD; //Running foreward
      UN    #tbRunningBack; //Running back
      UN    #tbRunningSlow; //Running slow
      UN    #tbRunningFast; //Running fast
      L     10; //Stopped
      SPB   COD2;
      L     0; //Undefined
COD2: T     LW    12; //States to OS

      UN    #tbRemoteLocal; //Local?
      L     256;
      SPB   COD3;
      U     #tbStateManual; //Manual?
      L     512;
      SPB   COD3;
      U     #tbStateAuto; // AUTO?
      L     1024;
      SPB   COD3;
      L     0;
COD3: L     LW    12; //Basic states
      +I    ;
      T     LW    12; //Combinate states to OS

NETWORK
TITLE = Store States in Record

      L     0; // Reset Commands OS
      T     #Motor3.CmdOS;
      T     #OSCOM; // Write Reset Back to I/O interface  added: 20060619 /Ho
      L     LW    10;
      T     #Motor3.AlarmOS; // Alarms to OS
      T     #OSALARM;
      L     LW    12;
      T     #Motor3.StatusOS; // States to OS
      T     #OSSTAT;
      L     LW    14;
      T     #Motor3.Status1; // Status stored
      L     LW    16;
      T     #Motor3.Status2; // Status stored
      L     LB    19;
      T     #Motor3.Status3; // Status stored
NETWORK
TITLE =Write record

      CALL "BLKMOV" (
           SRCBLK                   := #Motor3,
           RET_VAL                  := #siFailWR,
           DSTBLK                   := #P_currentRecord);

END_FUNCTION_BLOCK

